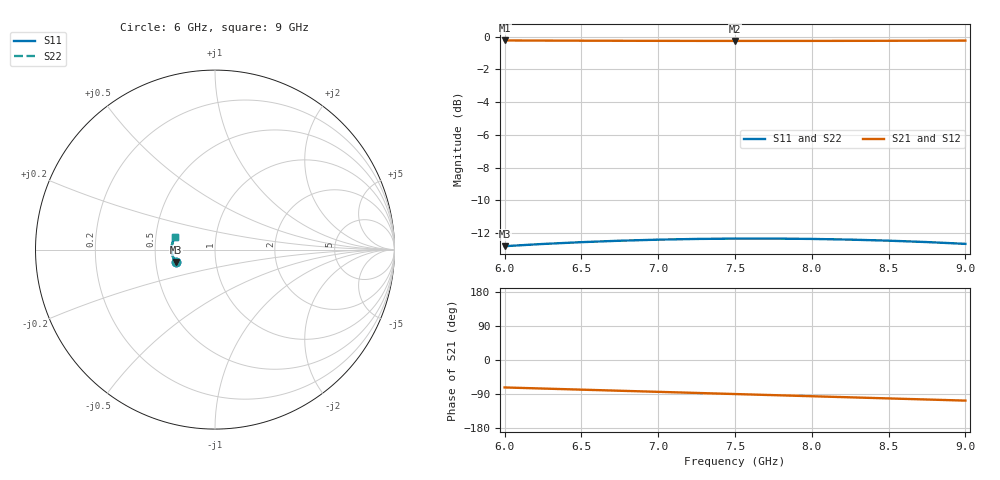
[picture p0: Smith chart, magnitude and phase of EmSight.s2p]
!AWR Design Environment (2469) Mon Oct 04 18:05:22 2004
!freq-unit  param-type  data-format  keyword  impedance-ohms
# GHz  S  MA  R  50
!Freq  MagS11  AngS11  MagS21  AngS21  MagS12  AngS12  MagS22  AngS22
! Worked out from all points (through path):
!   13 points, 6 GHz to 9 GHz, reference 50 ohm
!   highest |S21| = -0.23 dB at 6 GHz (marker M1); lowest = -0.3 dB at 7.5 GHz (marker M2)
!   group delay of S21, straight-line fit = 32.1 ps
!   lowest |S11| = -12.8 dB at 6 GHz (marker M3), VSWR 1.60, Z = 31.8 - j4.65 ohm
!   |S11| at or under -10 dB: start of sweep to end of sweep
!   |S22| runs from -12.8 to -12.3 dB; largest |S21 - S12| = 0
6  0.2294 -162.4  0.9733 -72.4  0.9733 -72.4  0.2294 -162.4
6.25  0.233 -165.3  0.9725 -75.3  0.9725 -75.3  0.233 -165.3
6.5  0.236 -168.2  0.9718 -78.2  0.9718 -78.2  0.236 -168.2
6.75  0.2384 -171.2  0.9712 -81.1  0.9712 -81.1  0.2384 -171.2
7  0.2402 -174.1  0.9707 -84.0  0.9707 -84.0  0.2402 -174.1
7.25  0.2414 -176.9  0.9704 -86.9  0.9704 -86.9  0.2414 -176.9
7.5  0.242 -179.8  0.9703 -89.8  0.9703 -89.8  0.242 -179.8
7.75  0.242 177.3  0.9703 -92.7  0.9703 -92.7  0.242 177.3
8  0.2414 174.4  0.9704 -95.6  0.9704 -95.6  0.2414 174.4
8.25  0.2402 171.5  0.9707 -98.5  0.9707 -98.5  0.2402 171.5
8.5  0.2385 168.6  0.9711 -101.4  0.9711 -101.4  0.2385 168.6
8.75  0.2361 165.7  0.9717 -104.3  0.9717 -104.3  0.2361 165.7
9  0.2332 162.8  0.9724 -107.2  0.9724 -107.2  0.2332 162.8
